DATA_BLOCK "IMAC_MOTOR2_I/O"
TITLE =
AUTHOR : Hottendo
FAMILY : IMAC
VERSION : 0.1


  STRUCT
   MOTOR2_001_ACOM : WORD ;	//MOTOR2 - Instance 001 : 'AUTO' Mode  Command Interface
   MOTOR2_001_STAT : WORD ;	//                        'AUTO' Mode  Status Interface
   MOTOR2_001_OSSTAT : WORD ;	//                        OS Status Word
   MOTOR2_001_OSALARM : WORD ;	//                        OS Alarm Word
   MOTOR2_001_OSCOM : WORD ;	//                        OS Command Interface
   MOTOR2_002_ACOM : WORD ;	//MOTOR2 - Instance 002 : 'AUTO' Mode  Command Interface
   MOTOR2_002_STAT : WORD ;	//                        'AUTO' Mode  Status Interface
   MOTOR2_002_OSSTAT : WORD ;	//                        OS Status Word
   MOTOR2_002_OSALARM : WORD ;	//                        OS Alarm Word
   MOTOR2_002_OSCOM : WORD ;	//                        OS Command Interface
   MOTOR2_003_ACOM : WORD ;	//MOTOR2 - Instance 003 : 'AUTO' Mode  Command Interface
   MOTOR2_003_STAT : WORD ;	//                        'AUTO' Mode  Status Interface
   MOTOR2_003_OSSTAT : WORD ;	//                        OS Status Word
   MOTOR2_003_OSALARM : WORD ;	//                        OS Alarm Word
   MOTOR2_003_OSCOM : WORD ;	//                        OS Command Interface
   MOTOR2_004_ACOM : WORD ;	//MOTOR2 - Instance 004 : 'AUTO' Mode  Command Interface
   MOTOR2_004_STAT : WORD ;	//                        'AUTO' Mode  Status Interface
   MOTOR2_004_OSSTAT : WORD ;	//                        OS Status Word
   MOTOR2_004_OSALARM : WORD ;	//                        OS Alarm Word
   MOTOR2_004_OSCOM : WORD ;	//                        OS Command Interface
   MOTOR2_005_ACOM : WORD ;	//MOTOR2 - Instance 005 : 'AUTO' Mode  Command Interface
   MOTOR2_005_STAT : WORD ;	//                        'AUTO' Mode  Status Interface
   MOTOR2_005_OSSTAT : WORD ;	//                        OS Status Word
   MOTOR2_005_OSALARM : WORD ;	//                        OS Alarm Word
   MOTOR2_005_OSCOM : WORD ;	//                        OS Command Interface
   MOTOR2_006_ACOM : WORD ;	//MOTOR2 - Instance 006 : 'AUTO' Mode  Command Interface
   MOTOR2_006_STAT : WORD ;	//                        'AUTO' Mode  Status Interface
   MOTOR2_006_OSSTAT : WORD ;	//                        OS Status Word
   MOTOR2_006_OSALARM : WORD ;	//                        OS Alarm Word
   MOTOR2_006_OSCOM : WORD ;	//                        OS Command Interface
   MOTOR2_007_ACOM : WORD ;	//MOTOR2 - Instance 007 : 'AUTO' Mode  Command Interface
   MOTOR2_007_STAT : WORD ;	//                        'AUTO' Mode  Status Interface
   MOTOR2_007_OSSTAT : WORD ;	//                        OS Status Word
   MOTOR2_007_OSALARM : WORD ;	//                        OS Alarm Word
   MOTOR2_007_OSCOM : WORD ;	//                        OS Command Interface
   MOTOR2_008_ACOM : WORD ;	//MOTOR2 - Instance 008 : 'AUTO' Mode  Command Interface
   MOTOR2_008_STAT : WORD ;	//                        'AUTO' Mode  Status Interface
   MOTOR2_008_OSSTAT : WORD ;	//                        OS Status Word
   MOTOR2_008_OSALARM : WORD ;	//                        OS Alarm Word
   MOTOR2_008_OSCOM : WORD ;	//                        OS Command Interface
   MOTOR2_009_ACOM : WORD ;	//MOTOR2 - Instance 009 : 'AUTO' Mode  Command Interface
   MOTOR2_009_STAT : WORD ;	//                        'AUTO' Mode  Status Interface
   MOTOR2_009_OSSTAT : WORD ;	//                        OS Status Word
   MOTOR2_009_OSALARM : WORD ;	//                        OS Alarm Word
   MOTOR2_009_OSCOM : WORD ;	//                        OS Command Interface
   MOTOR2_010_ACOM : WORD ;	//MOTOR2 - Instance 010 : 'AUTO' Mode  Command Interface
   MOTOR2_010_STAT : WORD ;	//                        'AUTO' Mode  Status Interface
   MOTOR2_010_OSSTAT : WORD ;	//                        OS Status Word
   MOTOR2_010_OSALARM : WORD ;	//                        OS Alarm Word
   MOTOR2_010_OSCOM : WORD ;	//                        OS Command Interface
   MOTOR2_011_ACOM : WORD ;	//MOTOR2 - Instance 011 : 'AUTO' Mode  Command Interface
   MOTOR2_011_STAT : WORD ;	//                        'AUTO' Mode  Status Interface
   MOTOR2_011_OSSTAT : WORD ;	//                        OS Status Word
   MOTOR2_011_OSALARM : WORD ;	//                        OS Alarm Word
   MOTOR2_011_OSCOM : WORD ;	//                        OS Command Interface
   MOTOR2_012_ACOM : WORD ;	//MOTOR2 - Instance 012 : 'AUTO' Mode  Command Interface
   MOTOR2_012_STAT : WORD ;	//                        'AUTO' Mode  Status Interface
   MOTOR2_012_OSSTAT : WORD ;	//                        OS Status Word
   MOTOR2_012_OSALARM : WORD ;	//                        OS Alarm Word
   MOTOR2_012_OSCOM : WORD ;	//                        OS Command Interface
   MOTOR2_013_ACOM : WORD ;	//MOTOR2 - Instance 013 : 'AUTO' Mode  Command Interface
   MOTOR2_013_STAT : WORD ;	//                        'AUTO' Mode  Status Interface
   MOTOR2_013_OSSTAT : WORD ;	//                        OS Status Word
   MOTOR2_013_OSALARM : WORD ;	//                        OS Alarm Word
   MOTOR2_013_OSCOM : WORD ;	//                        OS Command Interface
   MOTOR2_014_ACOM : WORD ;	//MOTOR2 - Instance 014 : 'AUTO' Mode  Command Interface
   MOTOR2_014_STAT : WORD ;	//                        'AUTO' Mode  Status Interface
   MOTOR2_014_OSSTAT : WORD ;	//                        OS Status Word
   MOTOR2_014_OSALARM : WORD ;	//                        OS Alarm Word
   MOTOR2_014_OSCOM : WORD ;	//                        OS Command Interface
   MOTOR2_015_ACOM : WORD ;	//MOTOR2 - Instance 015 : 'AUTO' Mode  Command Interface
   MOTOR2_015_STAT : WORD ;	//                        'AUTO' Mode  Status Interface
   MOTOR2_015_OSSTAT : WORD ;	//                        OS Status Word
   MOTOR2_015_OSALARM : WORD ;	//                        OS Alarm Word
   MOTOR2_015_OSCOM : WORD ;	//                        OS Command Interface
   MOTOR2_016_ACOM : WORD ;	//MOTOR2 - Instance 016 : 'AUTO' Mode  Command Interface
   MOTOR2_016_STAT : WORD ;	//                        'AUTO' Mode  Status Interface
   MOTOR2_016_OSSTAT : WORD ;	//                        OS Status Word
   MOTOR2_016_OSALARM : WORD ;	//                        OS Alarm Word
   MOTOR2_016_OSCOM : WORD ;	//                        OS Command Interface
   MOTOR2_017_ACOM : WORD ;	//MOTOR2 - Instance 017 : 'AUTO' Mode  Command Interface
   MOTOR2_017_STAT : WORD ;	//                        'AUTO' Mode  Status Interface
   MOTOR2_017_OSSTAT : WORD ;	//                        OS Status Word
   MOTOR2_017_OSALARM : WORD ;	//                        OS Alarm Word
   MOTOR2_017_OSCOM : WORD ;	//                        OS Command Interface
   MOTOR2_018_ACOM : WORD ;	//MOTOR2 - Instance 018 : 'AUTO' Mode  Command Interface
   MOTOR2_018_STAT : WORD ;	//                        'AUTO' Mode  Status Interface
   MOTOR2_018_OSSTAT : WORD ;	//                        OS Status Word
   MOTOR2_018_OSALARM : WORD ;	//                        OS Alarm Word
   MOTOR2_018_OSCOM : WORD ;	//                        OS Command Interface
   MOTOR2_019_ACOM : WORD ;	//MOTOR2 - Instance 019 : 'AUTO' Mode  Command Interface
   MOTOR2_019_STAT : WORD ;	//                        'AUTO' Mode  Status Interface
   MOTOR2_019_OSSTAT : WORD ;	//                        OS Status Word
   MOTOR2_019_OSALARM : WORD ;	//                        OS Alarm Word
   MOTOR2_019_OSCOM : WORD ;	//                        OS Command Interface
   MOTOR2_020_ACOM : WORD ;	//MOTOR2 - Instance 020 : 'AUTO' Mode  Command Interface
   MOTOR2_020_STAT : WORD ;	//                        'AUTO' Mode  Status Interface
   MOTOR2_020_OSSTAT : WORD ;	//                        OS Status Word
   MOTOR2_020_OSALARM : WORD ;	//                        OS Alarm Word
   MOTOR2_020_OSCOM : WORD ;	//                        OS Command Interface
   MOTOR2_021_ACOM : WORD ;	//MOTOR2 - Instance 021 : 'AUTO' Mode  Command Interface
   MOTOR2_021_STAT : WORD ;	//                        'AUTO' Mode  Status Interface
   MOTOR2_021_OSSTAT : WORD ;	//                        OS Status Word
   MOTOR2_021_OSALARM : WORD ;	//                        OS Alarm Word
   MOTOR2_021_OSCOM : WORD ;	//                        OS Command Interface
   MOTOR2_022_ACOM : WORD ;	//MOTOR2 - Instance 022 : 'AUTO' Mode  Command Interface
   MOTOR2_022_STAT : WORD ;	//                        'AUTO' Mode  Status Interface
   MOTOR2_022_OSSTAT : WORD ;	//                        OS Status Word
   MOTOR2_022_OSALARM : WORD ;	//                        OS Alarm Word
   MOTOR2_022_OSCOM : WORD ;	//                        OS Command Interface
   MOTOR2_023_ACOM : WORD ;	//MOTOR2 - Instance 023 : 'AUTO' Mode  Command Interface
   MOTOR2_023_STAT : WORD ;	//                        'AUTO' Mode  Status Interface
   MOTOR2_023_OSSTAT : WORD ;	//                        OS Status Word
   MOTOR2_023_OSALARM : WORD ;	//                        OS Alarm Word
   MOTOR2_023_OSCOM : WORD ;	//                        OS Command Interface
   MOTOR2_024_ACOM : WORD ;	//MOTOR2 - Instance 024 : 'AUTO' Mode  Command Interface
   MOTOR2_024_STAT : WORD ;	//                        'AUTO' Mode  Status Interface
   MOTOR2_024_OSSTAT : WORD ;	//                        OS Status Word
   MOTOR2_024_OSALARM : WORD ;	//                        OS Alarm Word
   MOTOR2_024_OSCOM : WORD ;	//                        OS Command Interface
   MOTOR2_025_ACOM : WORD ;	//MOTOR2 - Instance 025 : 'AUTO' Mode  Command Interface
   MOTOR2_025_STAT : WORD ;	//                        'AUTO' Mode  Status Interface
   MOTOR2_025_OSSTAT : WORD ;	//                        OS Status Word
   MOTOR2_025_OSALARM : WORD ;	//                        OS Alarm Word
   MOTOR2_025_OSCOM : WORD ;	//                        OS Command Interface
  END_STRUCT ;
BEGIN
   MOTOR2_001_ACOM := W#16#0;
   MOTOR2_001_STAT := W#16#0;
   MOTOR2_001_OSSTAT := W#16#0;
   MOTOR2_001_OSALARM := W#16#0;
   MOTOR2_001_OSCOM := W#16#0;
   MOTOR2_002_ACOM := W#16#0;
   MOTOR2_002_STAT := W#16#0;
   MOTOR2_002_OSSTAT := W#16#0;
   MOTOR2_002_OSALARM := W#16#0;
   MOTOR2_002_OSCOM := W#16#0;
   MOTOR2_003_ACOM := W#16#0;
   MOTOR2_003_STAT := W#16#0;
   MOTOR2_003_OSSTAT := W#16#0;
   MOTOR2_003_OSALARM := W#16#0;
   MOTOR2_003_OSCOM := W#16#0;
   MOTOR2_004_ACOM := W#16#0;
   MOTOR2_004_STAT := W#16#0;
   MOTOR2_004_OSSTAT := W#16#0;
   MOTOR2_004_OSALARM := W#16#0;
   MOTOR2_004_OSCOM := W#16#0;
   MOTOR2_005_ACOM := W#16#0;
   MOTOR2_005_STAT := W#16#0;
   MOTOR2_005_OSSTAT := W#16#0;
   MOTOR2_005_OSALARM := W#16#0;
   MOTOR2_005_OSCOM := W#16#0;
   MOTOR2_006_ACOM := W#16#0;
   MOTOR2_006_STAT := W#16#0;
   MOTOR2_006_OSSTAT := W#16#0;
   MOTOR2_006_OSALARM := W#16#0;
   MOTOR2_006_OSCOM := W#16#0;
   MOTOR2_007_ACOM := W#16#0;
   MOTOR2_007_STAT := W#16#0;
   MOTOR2_007_OSSTAT := W#16#0;
   MOTOR2_007_OSALARM := W#16#0;
   MOTOR2_007_OSCOM := W#16#0;
   MOTOR2_008_ACOM := W#16#0;
   MOTOR2_008_STAT := W#16#0;
   MOTOR2_008_OSSTAT := W#16#0;
   MOTOR2_008_OSALARM := W#16#0;
   MOTOR2_008_OSCOM := W#16#0;
   MOTOR2_009_ACOM := W#16#0;
   MOTOR2_009_STAT := W#16#0;
   MOTOR2_009_OSSTAT := W#16#0;
   MOTOR2_009_OSALARM := W#16#0;
   MOTOR2_009_OSCOM := W#16#0;
   MOTOR2_010_ACOM := W#16#0;
   MOTOR2_010_STAT := W#16#0;
   MOTOR2_010_OSSTAT := W#16#0;
   MOTOR2_010_OSALARM := W#16#0;
   MOTOR2_010_OSCOM := W#16#0;
   MOTOR2_011_ACOM := W#16#0;
   MOTOR2_011_STAT := W#16#0;
   MOTOR2_011_OSSTAT := W#16#0;
   MOTOR2_011_OSALARM := W#16#0;
   MOTOR2_011_OSCOM := W#16#0;
   MOTOR2_012_ACOM := W#16#0;
   MOTOR2_012_STAT := W#16#0;
   MOTOR2_012_OSSTAT := W#16#0;
   MOTOR2_012_OSALARM := W#16#0;
   MOTOR2_012_OSCOM := W#16#0;
   MOTOR2_013_ACOM := W#16#0;
   MOTOR2_013_STAT := W#16#0;
   MOTOR2_013_OSSTAT := W#16#0;
   MOTOR2_013_OSALARM := W#16#0;
   MOTOR2_013_OSCOM := W#16#0;
   MOTOR2_014_ACOM := W#16#0;
   MOTOR2_014_STAT := W#16#0;
   MOTOR2_014_OSSTAT := W#16#0;
   MOTOR2_014_OSALARM := W#16#0;
   MOTOR2_014_OSCOM := W#16#0;
   MOTOR2_015_ACOM := W#16#0;
   MOTOR2_015_STAT := W#16#0;
   MOTOR2_015_OSSTAT := W#16#0;
   MOTOR2_015_OSALARM := W#16#0;
   MOTOR2_015_OSCOM := W#16#0;
   MOTOR2_016_ACOM := W#16#0;
   MOTOR2_016_STAT := W#16#0;
   MOTOR2_016_OSSTAT := W#16#0;
   MOTOR2_016_OSALARM := W#16#0;
   MOTOR2_016_OSCOM := W#16#0;
   MOTOR2_017_ACOM := W#16#0;
   MOTOR2_017_STAT := W#16#0;
   MOTOR2_017_OSSTAT := W#16#0;
   MOTOR2_017_OSALARM := W#16#0;
   MOTOR2_017_OSCOM := W#16#0;
   MOTOR2_018_ACOM := W#16#0;
   MOTOR2_018_STAT := W#16#0;
   MOTOR2_018_OSSTAT := W#16#0;
   MOTOR2_018_OSALARM := W#16#0;
   MOTOR2_018_OSCOM := W#16#0;
   MOTOR2_019_ACOM := W#16#0;
   MOTOR2_019_STAT := W#16#0;
   MOTOR2_019_OSSTAT := W#16#0;
   MOTOR2_019_OSALARM := W#16#0;
   MOTOR2_019_OSCOM := W#16#0;
   MOTOR2_020_ACOM := W#16#0;
   MOTOR2_020_STAT := W#16#0;
   MOTOR2_020_OSSTAT := W#16#0;
   MOTOR2_020_OSALARM := W#16#0;
   MOTOR2_020_OSCOM := W#16#0;
   MOTOR2_021_ACOM := W#16#0;
   MOTOR2_021_STAT := W#16#0;
   MOTOR2_021_OSSTAT := W#16#0;
   MOTOR2_021_OSALARM := W#16#0;
   MOTOR2_021_OSCOM := W#16#0;
   MOTOR2_022_ACOM := W#16#0;
   MOTOR2_022_STAT := W#16#0;
   MOTOR2_022_OSSTAT := W#16#0;
   MOTOR2_022_OSALARM := W#16#0;
   MOTOR2_022_OSCOM := W#16#0;
   MOTOR2_023_ACOM := W#16#0;
   MOTOR2_023_STAT := W#16#0;
   MOTOR2_023_OSSTAT := W#16#0;
   MOTOR2_023_OSALARM := W#16#0;
   MOTOR2_023_OSCOM := W#16#0;
   MOTOR2_024_ACOM := W#16#0;
   MOTOR2_024_STAT := W#16#0;
   MOTOR2_024_OSSTAT := W#16#0;
   MOTOR2_024_OSALARM := W#16#0;
   MOTOR2_024_OSCOM := W#16#0;
   MOTOR2_025_ACOM := W#16#0;
   MOTOR2_025_STAT := W#16#0;
   MOTOR2_025_OSSTAT := W#16#0;
   MOTOR2_025_OSALARM := W#16#0;
   MOTOR2_025_OSCOM := W#16#0;
END_DATA_BLOCK

